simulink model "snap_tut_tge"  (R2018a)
settings: Solver=VariableStepDiscrete  StartTime=0.0  StopTime=50000  RelTol=1e-3
undefined symbols (not defined in the file): bad_frame, Bit, Both, bram, c, cnt_rst, core_rst, d, data, data_in, eof, eof_in, Falling, hex2dec, ip, ip_in, led, led_rx, led_tx, led_up, link_up, Location, Lower, Minimum_Area, notused, out, overrun, reg, Rising, ROACH2, sfp, SNAP, tx_full, tx_over, Unsigned, Upper, valid, valid_in, Width, xc7k160t
libraries: xbsIndex_r4 x1201, casper_library_misc x9, xps_library x5
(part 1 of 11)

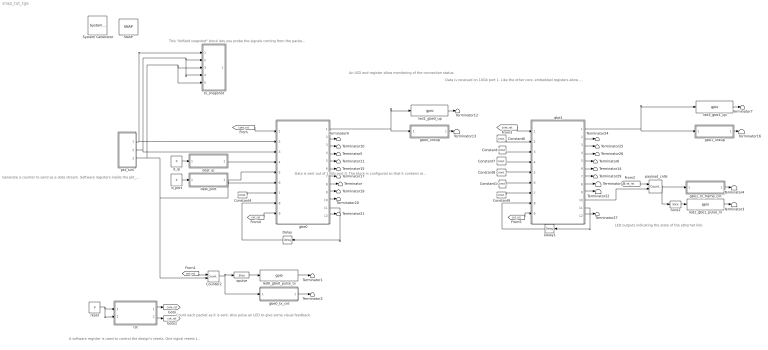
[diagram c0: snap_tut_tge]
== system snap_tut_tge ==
  note: A software register is used to control the design's resets. One signal resets the cores, the other resets the various status counters.
  note: This "bitfield snapshot" block lets you probe the signals coming from the packet simulator Using the valid signal to drive "we" and the end of frame to drive "trig" means that we can capture data starting at the beginning of a packet
  note: An LED and register allow monitoring of the connection status.
  note: Count each packet as it is sent. Also pulse an LED to give some visual feedback.
  note: LED outputs indicating the state of the ethernet link.
  note: Data is sent out of 10Gb port 0. The block is configured so that it contains all sorts of internal debug logic to count the packet rates out of, and in to, the core. The casperfpga control software knows the layout of registers inside this block, which makes it easy to grab status information
  note: Generate a counter to send as a data stream. Software registers inside the pkt_sim block allow packet sizes and counter period to be set dynamically at runtime.
  note: Data is received on 10Gb port 1. Like the other core, embedded registers allow status monitoring
  " System Generator" : xbsIndex_r4/ System Generator  Tag=genX  xilinxfamily=kintex7  part=xc7k160t  speed=-2  package=ffg676  synthesis_tool=XST  clock_wrapper=Clock Enables  directory=/home/jackh/mergeymcmergeface/tutorials_devel2/vivado/snap/tut_tge/snap_tut_tge/sysgen  proj_type=Vivado  Synth_file=Vivado Synthesis Defaults  Impl_file=Vivado Implementation Defaults  testbench=off  simulink_period=1  sysclk_period=10  dcm_input_clock_period=10  incr_netlist=off  trim_vbits=Everywhere in SubSystem  dbl_ovrd=According to Block Masks  core_generation=According to Block Masks  run_coregen=off  deprecated_control=off  eval_field=0  block_type=sysgen
  Constant : xbsIndex_r4/Constant  const=0  gui_display_data_type=Boolean  arith_type=Boolean  n_bits=16  bin_pt=14  preci_type=Single  exp_width=8  frac_width=24  explicit_period=on  period=1  equ=P=C  opselect=C  inp2=PCIN>>17  opr=+  inp1=P  carry=CIN  dbl_ovrd=off  block_type=constant
  Constant1 : xbsIndex_r4/Constant  const=0  gui_display_data_type=Boolean  arith_type=Boolean  n_bits=16  bin_pt=14  preci_type=Single  exp_width=8  frac_width=24  explicit_period=on  period=1  equ=P=C  opselect=C  inp2=PCIN>>17  opr=+  inp1=P  carry=CIN  dbl_ovrd=off  block_type=constant
  Constant4 : xbsIndex_r4/Constant  const=1  gui_display_data_type=Fixed-point  arith_type=Boolean  n_bits=1  bin_pt=0  preci_type=Single  exp_width=8  frac_width=24  explicit_period=on  period=1  equ=P=C  opselect=C  inp2=PCIN>>17  opr=+  inp1=P  carry=CIN  dbl_ovrd=off  block_type=constant
  Constant6 : xbsIndex_r4/Constant  const=0  gui_display_data_type=Fixed-point  arith_type=Unsigned  n_bits=64  bin_pt=0  preci_type=Single  exp_width=8  frac_width=24  explicit_period=on  period=1  equ=P=C  opselect=C  inp2=PCIN>>17  opr=+  inp1=P  carry=CIN  dbl_ovrd=off  block_type=constant
  Constant7 : xbsIndex_r4/Constant  const=0  gui_display_data_type=Fixed-point  arith_type=Unsigned  n_bits=32  bin_pt=0  preci_type=Single  exp_width=8  frac_width=24  explicit_period=on  period=1  equ=P=C  opselect=C  inp2=PCIN>>17  opr=+  inp1=P  carry=CIN  dbl_ovrd=off  block_type=constant
  Constant8 : xbsIndex_r4/Constant  const=0  gui_display_data_type=Fixed-point  arith_type=Unsigned  n_bits=16  bin_pt=0  preci_type=Single  exp_width=8  frac_width=24  explicit_period=on  period=1  equ=P=C  opselect=C  inp2=PCIN>>17  opr=+  inp1=P  carry=CIN  dbl_ovrd=off  block_type=constant
  Constant9 : xbsIndex_r4/Constant  const=1  gui_display_data_type=Fixed-point  arith_type=Boolean  n_bits=1  bin_pt=0  preci_type=Single  exp_width=8  frac_width=24  explicit_period=on  period=1  equ=P=C  opselect=C  inp2=PCIN>>17  opr=+  inp1=P  carry=CIN  dbl_ovrd=off  block_type=constant
  Counter2 : xbsIndex_r4/Counter  cnt_type=Free Running  cnt_to=Inf  operation=Up  start_count=0  cnt_by_val=1  arith_type=Unsigned  n_bits=32  bin_pt=0  load_pin=off  rst=on  en=on  explicit_period=on  period=1  use_behavioral_HDL=off  implementation=Fabric  dbl_ovrd=off  block_type=counter
  Delay : xbsIndex_r4/Delay  rst=off  infoeditControl=Selection of Reset will increase slice count due to use of real FFs and instead of SRLs  en=off  latency=1  reg_retiming=on  dbl_ovrd=off  block_type=delay
  Delay1 : xbsIndex_r4/Delay  rst=off  infoeditControl=Selection of Reset will increase slice count due to use of real FFs and instead of SRLs  en=off  latency=1  reg_retiming=on  dbl_ovrd=off  block_type=delay
  SNAP : xps_library/Platforms/SNAP  Tag=xps:xsg  hw_sys=SNAP:xc7k160t  clk_src=sys_clk  clk_rate=100  use_microblaze=off  sample_period=1  synthesis_tool=XST
  Slice2 : xbsIndex_r4/Slice  nbits=1  boolean_output=on  mode=Lower Bit Location + Width  bit1=0  base1=MSB of Input  bit0=27-12  base0=LSB of Input  dbl_ovrd=off  block_type=slice
  Terminator{,1..7,9..22,24..27,29} (27 alike) : Terminator
  d_ip : Constant  Value=0
  d_port : Constant  Value=0
  dest_ip : Subsystem  Tag=xps:sw_reg  AncestorBlock=xps_library/Memory/software_register  mask(swreg){io_dir=From Processor, io_delay=0, init_val=0, sample_period=1, names=reg, bitwidths=32, bin_pts=0, arith_types=0, sim_port=on, show_format=off}
      mask prompts: io_dir "I/O direction"; io_delay "I/O delay"; init_val "Initial Value"; sample_period "Sample period"; names "Bitfield names [msb...lsb]"; bitwidths "Bitfield widths"; bin_pts "Bitfield binary pts"; arith_types "Bitfield types, ufix=0, fix=1, bool=2"; sim_port "Provide sim input/output?"; show_format "Print format string?"
      mask help: A 32-bit software-accessible register. Can be divided into bitfields of varying widths and types using the fields in the block mask.
      mask init:
      | swreg_init(gcb)
  dest_port : Subsystem  Tag=xps:sw_reg  AncestorBlock=xps_library/Memory/software_register  mask(swreg){io_dir=From Processor, io_delay=0, init_val=0, sample_period=1, names=reg, bitwidths=16, bin_pts=0, arith_types=0, sim_port=on, show_format=off}
      mask prompts: io_dir "I/O direction"; io_delay "I/O delay"; init_val "Initial Value"; sample_period "Sample period"; names "Bitfield names [msb...lsb]"; bitwidths "Bitfield widths"; bin_pts "Bitfield binary pts"; arith_types "Bitfield types, ufix=0, fix=1, bool=2"; sim_port "Provide sim input/output?"; show_format "Print format string?"
      mask help: A 32-bit software-accessible register. Can be divided into bitfields of varying widths and types using the fields in the block mask.
      mask init:
      | swreg_init(gcb)
  gbe0 : Subsystem  Tag=xps:ten_gbe  AncestorBlock=xps_library/IO/ten_gbe  mask(ten_gbe){flavour=sfp+, slot=0, port_r1=0, port_r2_cx4=0, port_r2_sfpp=0, rx_dist_ram=off, large_frames=on, show_param=off, pre_emph_r2=1.07, pre_emph=3, post_emph_r2=0.18, rxeqmix_r2=7, swing_r2=940, swing=800, fab_en=on, fab_mac=hex2dec('123456780000'), fab_ip=192*(2^24) + 168*(2^16) + 5*(2^8) + 20*(2^0), fab_udp=10000, fab_gate=1, cpu_rx_en=on, cpu_tx_en=on, ttl=hex2dec('FF'), promisc_mode=off, debug_ctr_width=32, txctr=on, txerrctr=off, txerrctr_len=100, txofctr=on, txfullctr=on, txvldctr=on, txsnaplen=8192, rxctr=on, rxerrctr=off, rxerrctr_len=100, rxofctr=on, rxbadctr=on, rxvldctr=on, rxeofctr=on, rxsnaplen=8192}
      mask prompts: flavour "Mezzanine card flavour"; slot "Card slot"; port_r1 "Port"; port_r2_cx4 "Port"; port_r2_sfpp "Port"; rx_dist_ram "Shallow RX Fifo (Beware overruns!)"; large_frames "Enable Large TX Frames (8k+512)"; show_param "---------------------- Show Implementation Parameters -----------------------------------------------------------------------------------"; pre_emph_r2 "Pre-emphasis (dB)"; pre_emph "Pre-emphasis"; post_emph_r2 "Post-emphasis (dB)"; rxeqmix_r2 "Receive equalisation"; swing_r2 "Driver Swing Control (mVppd)"; swing "Differential swing"; fab_en "Enable fabric on startup"; fab_mac "Fabric MAC Address"; fab_ip "Fabric IP Address"; fab_udp "Fabric UDP Port"; fab_gate "Fabric Gateway"; cpu_rx_en "Enable CPU RX"; cpu_tx_en "Enable CPU TX"; promisc_mode "Promiscuous mode"; debug_ctr_width "Debug counter width"; txctr "TX - core_txctr"; txerrctr "TX packet length error - core_txerrctr"; txerrctr_len "-- expected TX packet length"; txofctr "TX overflow - core_txofctr"; txfullctr "TX full - core_txfullctr"; txvldctr "TX valid cycle - core_txvldctr"; txsnaplen "TX snapshot length"; rxctr "RX - core_rxctr"; rxerrctr "RX packet length error - core_rxerrctr"; rxerrctr_len "-- expected RX packet length"; rxofctr "RX overflow - core_rxofctr"; rxbadctr "RX bad - core_rxbadctr"; rxvldctr "RX valid cycle - core_rxvldctr"; rxeofctr "RX eof - core_rxeofctr"; rxsnaplen "RX snapshot length"
      mask help: This block sends and receives UDP frames (packets). It accepts a 64 bit wide data stream with user-determined frame breaks. The data stream is wrapped in a UDP frame for transmission. Incoming UDP packets are unwrapped and the data presented as a 64 bit wide stream.
      mask init:
      | temp = eval(get_param(gcb, 'debug_ctr_width'));
      | if temp <= 0,
      |     error('Debug counters cannot be ltoet zero.');
      | end
      | tengbe_mask(gcb)
  gbe0_linkup : Subsystem  Tag=xps:sw_reg  AncestorBlock=xps_library/Memory/software_register  mask(swreg){io_dir=To Processor, io_delay=0, init_val=0, sample_period=1, names=reg, bitwidths=1, bin_pts=0, arith_types=2, sim_port=on, show_format=off}
      mask prompts: io_dir "I/O direction"; io_delay "I/O delay"; init_val "Initial Value"; sample_period "Sample period"; names "Bitfield names [msb...lsb]"; bitwidths "Bitfield widths"; bin_pts "Bitfield binary pts"; arith_types "Bitfield types, ufix=0, fix=1, bool=2"; sim_port "Provide sim input/output?"; show_format "Print format string?"
      mask help: A 32-bit software-accessible register. Can be divided into bitfields of varying widths and types using the fields in the block mask.
      mask init:
      | swreg_init(gcb)
  gbe0_tx_cnt : Subsystem  Tag=xps:sw_reg  AncestorBlock=xps_library/Memory/software_register  mask(swreg){io_dir=To Processor, io_delay=0, init_val=0, sample_period=1, names=reg, bitwidths=32, bin_pts=0, arith_types=0, sim_port=on, show_format=off}
      mask prompts: io_dir "I/O direction"; io_delay "I/O delay"; init_val "Initial Value"; sample_period "Sample period"; names "Bitfield names [msb...lsb]"; bitwidths "Bitfield widths"; bin_pts "Bitfield binary pts"; arith_types "Bitfield types, ufix=0, fix=1, bool=2"; sim_port "Provide sim input/output?"; show_format "Print format string?"
      mask help: A 32-bit software-accessible register. Can be divided into bitfields of varying widths and types using the fields in the block mask.
      mask init:
      | swreg_init(gcb)
  gbe1 : Subsystem  Tag=xps:ten_gbe  AncestorBlock=xps_library/IO/ten_gbe  mask(ten_gbe){flavour=sfp+, slot=0, port_r1=1, port_r2_cx4=0, port_r2_sfpp=0, rx_dist_ram=off, large_frames=on, show_param=on, pre_emph_r2=1.07, pre_emph=3, post_emph_r2=0.18, rxeqmix_r2=7, swing_r2=940, swing=800, fab_en=on, fab_mac=hex2dec('123456780001'), fab_ip=192*(2^24) + 168*(2^16) + 5*(2^8) + 21*(2^0), fab_udp=10000, fab_gate=1, cpu_rx_en=on, cpu_tx_en=on, ttl=hex2dec('FF'), promisc_mode=off, debug_ctr_width=32, txctr=on, txerrctr=off, txerrctr_len=100, txofctr=on, txfullctr=on, txvldctr=on, txsnaplen=8192, rxctr=on, rxerrctr=off, rxerrctr_len=100, rxofctr=on, rxbadctr=on, rxvldctr=on, rxeofctr=on, rxsnaplen=8192}
      mask prompts: flavour "Mezzanine card flavour"; slot "Card slot"; port_r1 "Port"; port_r2_cx4 "Port"; port_r2_sfpp "Port"; rx_dist_ram "Shallow RX Fifo (Beware overruns!)"; large_frames "Enable Large TX Frames (8k+512)"; show_param "---------------------- Show Implementation Parameters -----------------------------------------------------------------------------------"; pre_emph_r2 "Pre-emphasis (dB)"; pre_emph "Pre-emphasis"; post_emph_r2 "Post-emphasis (dB)"; rxeqmix_r2 "Receive equalisation"; swing_r2 "Driver Swing Control (mVppd)"; swing "Differential swing"; fab_en "Enable fabric on startup"; fab_mac "Fabric MAC Address"; fab_ip "Fabric IP Address"; fab_udp "Fabric UDP Port"; fab_gate "Fabric Gateway"; cpu_rx_en "Enable CPU RX"; cpu_tx_en "Enable CPU TX"; promisc_mode "Promiscuous mode"; debug_ctr_width "Debug counter width"; txctr "TX - core_txctr"; txerrctr "TX packet length error - core_txerrctr"; txerrctr_len "-- expected TX packet length"; txofctr "TX overflow - core_txofctr"; txfullctr "TX full - core_txfullctr"; txvldctr "TX valid cycle - core_txvldctr"; txsnaplen "TX snapshot length"; rxctr "RX - core_rxctr"; rxerrctr "RX packet length error - core_rxerrctr"; rxerrctr_len "-- expected RX packet length"; rxofctr "RX overflow - core_rxofctr"; rxbadctr "RX bad - core_rxbadctr"; rxvldctr "RX valid cycle - core_rxvldctr"; rxeofctr "RX eof - core_rxeofctr"; rxsnaplen "RX snapshot length"
      mask help: This block sends and receives UDP frames (packets). It accepts a 64 bit wide data stream with user-determined frame breaks. The data stream is wrapped in a UDP frame for transmission. Incoming UDP packets are unwrapped and the data presented as a 64 bit wide stream.
      mask init:
      | temp = eval(get_param(gcb, 'debug_ctr_width'));
      | if temp <= 0,
      |     error('Debug counters cannot be ltoet zero.');
      | end
      | tengbe_mask(gcb)
  gbe1_linkup : Subsystem  Tag=xps:sw_reg  AncestorBlock=xps_library/Memory/software_register  mask(swreg){io_dir=To Processor, io_delay=0, init_val=0, sample_period=1, names=reg, bitwidths=1, bin_pts=0, arith_types=2, sim_port=on, show_format=off}
      mask prompts: io_dir "I/O direction"; io_delay "I/O delay"; init_val "Initial Value"; sample_period "Sample period"; names "Bitfield names [msb...lsb]"; bitwidths "Bitfield widths"; bin_pts "Bitfield binary pts"; arith_types "Bitfield types, ufix=0, fix=1, bool=2"; sim_port "Provide sim input/output?"; show_format "Print format string?"
      mask help: A 32-bit software-accessible register. Can be divided into bitfields of varying widths and types using the fields in the block mask.
      mask init:
      | swreg_init(gcb)
  gbe1_rx_frame_cnt : Subsystem  Tag=xps:sw_reg  AncestorBlock=xps_library/Memory/software_register  mask(swreg){io_dir=To Processor, io_delay=0, init_val=0, sample_period=1, names=reg, bitwidths=32, bin_pts=0, arith_types=0, sim_port=on, show_format=off}
      mask prompts: io_dir "I/O direction"; io_delay "I/O delay"; init_val "Initial Value"; sample_period "Sample period"; names "Bitfield names [msb...lsb]"; bitwidths "Bitfield widths"; bin_pts "Bitfield binary pts"; arith_types "Bitfield types, ufix=0, fix=1, bool=2"; sim_port "Provide sim input/output?"; show_format "Print format string?"
      mask help: A 32-bit software-accessible register. Can be divided into bitfields of varying widths and types using the fields in the block mask.
      mask init:
      | swreg_init(gcb)
  led0_gbe0_pulse_tx : xps_library/IO/gpio  Tag=xps:gpio  io_group_params_forwarded=on  io_group=ROACH2:led  io_group_real=led  io_group_custom=0  io_dir=out  arith_type=Boolean  bitwidth=1  bin_pt=0  bit_index=0  sample_period=1  use_single_ended=off  use_ddr=off  reg_iob=on  reg_clk_phase=0  termination=None
  led1_gbe0_up : xps_library/IO/gpio  Tag=xps:gpio  io_group_params_forwarded=on  io_group=ROACH2:led  io_group_real=led  io_group_custom=0  io_dir=out  arith_type=Boolean  bitwidth=1  bin_pt=0  bit_index=1  sample_period=1  use_single_ended=off  use_ddr=off  reg_iob=on  reg_clk_phase=0  termination=None
  led2_gbe1_pulse_rx : xps_library/IO/gpio  Tag=xps:gpio  io_group_params_forwarded=on  io_group=ROACH2:led  io_group_real=led  io_group_custom=0  io_dir=out  arith_type=Boolean  bitwidth=1  bin_pt=0  bit_index=2  sample_period=1  use_single_ended=off  use_ddr=off  reg_iob=off  reg_clk_phase=0  termination=None
  led3_gbe1_up : xps_library/IO/gpio  Tag=xps:gpio  io_group_params_forwarded=on  io_group=ROACH2:led  io_group_real=led  io_group_custom=0  io_dir=out  arith_type=Boolean  bitwidth=2  bin_pt=0  bit_index=3  sample_period=1  use_single_ended=off  use_ddr=off  reg_iob=on  reg_clk_phase=0  termination=None
  payload_cnt6 : xbsIndex_r4/Counter  cnt_type=Free Running  cnt_to=0  operation=Up  start_count=0  cnt_by_val=1  arith_type=Unsigned  n_bits=32  bin_pt=0  load_pin=off  rst=on  en=on  explicit_period=on  period=1  use_behavioral_HDL=off  implementation=Fabric  use_rpm=on  dbl_ovrd=off  block_type=counter
  pkt_sim : Subsystem
  reset : Constant  Value=0
  rst : Subsystem  Tag=xps:sw_reg  AncestorBlock=xps_library/Memory/software_register  mask(swreg){io_dir=From Processor, io_delay=0, init_val=0, sample_period=1, names=[core_rst cnt_rst], bitwidths=[1 1], bin_pts=0, arith_types=[2 2], sim_port=on, show_format=off}
      mask prompts: io_dir "I/O direction"; io_delay "I/O delay"; init_val "Initial Value"; sample_period "Sample period"; names "Bitfield names [msb...lsb]"; bitwidths "Bitfield widths"; bin_pts "Bitfield binary pts"; arith_types "Bitfield types, ufix=0, fix=1, bool=2"; sim_port "Provide sim input/output?"; show_format "Print format string?"
      mask help: A 32-bit software-accessible register. Can be divided into bitfields of varying widths and types using the fields in the block mask.
      mask init:
      | swreg_init(gcb)
  spulse : xbsIndex_r4/Slice  nbits=1  boolean_output=on  mode=Lower Bit Location + Width  bit1=0  base1=MSB of Input  bit0=27-12  base0=LSB of Input  dbl_ovrd=off  block_type=slice
  tx_snapshot : Subsystem  Tag=casper:bitsnap  AncestorBlock=casper_library_scopes/bitfield_snapshot  mask(bitsnap){io_names=[data valid eof], io_widths=[64 1 1], io_bps=[0 0 0], io_types=[0 2 2], show_format=on, snap_storage=bram, snap_dram_dimm=2, snap_dram_clock=250, snap_nsamples=12, snap_data_width=128, snap_offset=off, snap_circap=off, snap_value=off, snap_ext_arm=off, snap_ext_circ=off, snap_provide_outputs=on, snap_use_dsp48=on, snap_delay=0, extra_names=[c d], extra_widths=[30 2], extra_bps=[0 0], extra_types=[0 0]}
      mask prompts: io_names "Names [msb...lsb]"; io_widths "Bitwidths [msb...lsb]"; io_bps "Binary pts [msb...lsb]"; io_types "Data types [msb...lsb], ufix=0, fix=1, bool=2"; show_format "Print format string?"; snap_storage "Storage medium"; snap_dram_dimm "DRAM dimm"; snap_dram_clock "DRAM clock rate"; snap_nsamples "Number of Samples (2^?)"; snap_data_width "Data width"; snap_offset "Start delay support"; snap_circap "Circular capture support"; snap_value "Extra value capture support"; snap_ext_arm "External arm support"; snap_ext_circ "External circular capture support"; snap_provide_outputs "Provide outputs"; snap_use_dsp48 "Use DSP48s to implement counters"; snap_delay "Pre-snapshot delay"; extra_names "Names [msb...lsb]"; extra_widths "Widths [msb...lsb]"; extra_bps "Binary pts [msb...lsb]"; extra_types "Data types [msb...lsb], ufix=0, fix=1, bool=2"
      mask help: A wrapped snapshot block. Allows specification of inputs to a snapblock word so the toolflow can automatically set up the scope. See documentation for snapshot for explanation of parameters.
      mask init:
      | bitsnap_init(gcb);
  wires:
  reset/1 -> rst/2(sim_2), rst/1(sim_1)
  rst/2(in_cnt_rst) -> [cnt_rst]
  rst/1(in_core_rst) -> [core_rst]
  dest_ip/1(in_reg) -> gbe0/4(tx_dest_ip)
  dest_port/1(in_reg) -> gbe0/5(tx_dest_port)
  d_ip/1 -> dest_ip/1(sim_1)
  d_port/1 -> dest_port/1(sim_1)
  [core_rst] -> gbe0/1(rst)
  pkt_sim/1(d_out) -> gbe0/2(tx_data), tx_snapshot/1(in_data)
  Constant4/1 -> gbe0/7(rx_ack)
  gbe0/11(rx_bad_frame) -> Delay/1
  gbe0/8(rx_source_ip) -> Terminator/1
  Delay/1 -> gbe0/8(rx_overrun_ack)
  spulse/1 -> led0_gbe0_pulse_tx/1
  Counter2/1 -> spulse/1, gbe0_tx_cnt/1(out_reg)
  [cnt_rst] -> Counter2/1
  led0_gbe0_pulse_tx/1 -> Terminator1/1
  gbe0_tx_cnt/1(sim_out) -> Terminator2/1
  gbe0_linkup/1(sim_out) -> Terminator13/1
  [cnt_rst] -> payload_cnt6/1
  Constant6/1 -> gbe1/2(tx_data)
  Constant/1 -> gbe1/3(tx_valid)
  Constant7/1 -> gbe1/4(tx_dest_ip)
  Constant8/1 -> gbe1/5(tx_dest_port)
  Constant1/1 -> gbe1/6(tx_end_of_frame)
  Constant9/1 -> gbe1/7(rx_ack)
  gbe1/11(rx_bad_frame) -> Delay1/1
  Delay1/1 -> gbe1/8(rx_overrun_ack)
  payload_cnt6/1 -> gbe1_rx_frame_cnt/1(out_reg), Slice2/1
  Slice2/1 -> led2_gbe1_pulse_rx/1
  [core_rst] -> gbe1/1(rst)
  gbe1_rx_frame_cnt/1(sim_out) -> Terminator4/1
  led2_gbe1_pulse_rx/1 -> Terminator3/1
  gbe1_linkup/1(sim_out) -> Terminator16/1
  gbe1/8(rx_source_ip) -> Terminator18/1
  gbe0/1(led_up) -> led1_gbe0_up/1, gbe0_linkup/1(out_reg)
  led1_gbe0_up/1 -> Terminator12/1
  led3_gbe1_up/1 -> Terminator7/1
  gbe1/1(led_up) -> gbe1_linkup/1(out_reg), led3_gbe1_up/1
  gbe0/2(led_rx) -> Terminator9/1
  gbe0/3(led_tx) -> Terminator10/1
  gbe0/5(tx_overflow) -> Terminator11/1
  gbe0/6(rx_data) -> Terminator15/1
  gbe0/7(rx_valid) -> Terminator17/1
  gbe0/9(rx_source_port) -> Terminator19/1
  gbe0/10(rx_end_of_frame) -> Terminator20/1
  gbe0/12(rx_overrun) -> Terminator21/1
  gbe1/2(led_rx) -> Terminator24/1
  gbe1/3(led_tx) -> Terminator25/1
  gbe1/4(tx_afull) -> Terminator26/1
  gbe1/12(rx_overrun) -> Terminator27/1
  [cnt_rst] -> gbe0/9(debug_rst)
  [cnt_rst] -> gbe1/9(debug_rst)
  gbe0/4(tx_afull) -> Terminator5/1
  gbe1/5(tx_overflow) -> Terminator6/1
  gbe1/6(rx_data) -> Terminator14/1
  gbe1/7(rx_valid) -> Terminator29/1
  gbe1/10(rx_end_of_frame) -> payload_cnt6/2
  gbe1/9(rx_source_port) -> Terminator22/1
  pkt_sim/3(eof) -> tx_snapshot/5(trig), tx_snapshot/3(in_eof), gbe0/6(tx_end_of_frame), Counter2/2
  pkt_sim/2(valid) -> gbe0/3(tx_valid), tx_snapshot/4(we), tx_snapshot/2(in_valid)

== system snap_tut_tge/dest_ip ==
  sim_1 : Inport
  convert1_1 : DataTypeConversion  OutDataTypeStr=fixdt('ufix32_En0')
  convert2_1 : DataTypeConversion  OutDataTypeStr=fixdt('ufix32_En0')  ConvertRealWorld=Stored Integer (SI)
  gain_1 : Gain
  io_delay : xbsIndex_r4/Delay  rst=off  infoeditControl=Selection of Reset will increase slice count due to use of real FFs and instead of SRLs  en=off  latency=0  reg_retiming=on  dbl_ovrd=off  block_type=delay
  reint1 : xbsIndex_r4/Reinterpret  force_arith_type=on  arith_type=Unsigned  force_bin_pt=on  bin_pt=0  block_type=reinterpret
  slice_reg : xbsIndex_r4/Slice  nbits=32  boolean_output=off  mode=Lower Bit Location + Width  bit1=0  base1=MSB of Input  bit0=0  base0=LSB of Input  dbl_ovrd=off  block_type=slice
  snap_tut_tge_dest_ip_user_data_out : xbsIndex_r4/Gateway In  gui_display_data_type=Fixed-point  arith_type=Unsigned  n_bits=32  bin_pt=0  preci_type=Single  exp_width=8  frac_width=24  rows=1  columns=1  quantization="Round  (unbiased: +/- Inf)"  overflow=Saturate  period=1  UseAsADC=off  ADCChannel='1'  interface=None  automatic_assignment=on  address_offset=hex2dec('00')  intf_name=''  intf_description=''  default_value=0  timing_constraint=None  locs_specified=off  LOCs={}  io_standard={}  inherit_from_input=off  hdl_port=on  dbl_ovrd=off  block_type=gatewayin
  in_reg : Outport
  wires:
  snap_tut_tge_dest_ip_user_data_out/1 -> io_delay/1
  sim_1/1 -> convert1_1/1
  convert1_1/1 -> convert2_1/1
  convert2_1/1 -> gain_1/1
  gain_1/1 -> snap_tut_tge_dest_ip_user_data_out/1
  io_delay/1 -> slice_reg/1
  slice_reg/1 -> reint1/1
  reint1/1 -> in_reg/1

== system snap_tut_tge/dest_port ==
  sim_1 : Inport
  convert1_1 : DataTypeConversion  OutDataTypeStr=fixdt('ufix16_En0')
  convert2_1 : DataTypeConversion  OutDataTypeStr=fixdt('ufix16_En0')  ConvertRealWorld=Stored Integer (SI)
  gain_1 : Gain
  io_delay : xbsIndex_r4/Delay  rst=off  infoeditControl=Selection of Reset will increase slice count due to use of real FFs and instead of SRLs  en=off  latency=0  reg_retiming=on  dbl_ovrd=off  block_type=delay
  reint1 : xbsIndex_r4/Reinterpret  force_arith_type=on  arith_type=Unsigned  force_bin_pt=on  bin_pt=0  block_type=reinterpret
  slice_reg : xbsIndex_r4/Slice  nbits=16  boolean_output=off  mode=Lower Bit Location + Width  bit1=0  base1=MSB of Input  bit0=0  base0=LSB of Input  dbl_ovrd=off  block_type=slice
  snap_tut_tge_dest_port_user_data_out : xbsIndex_r4/Gateway In  gui_display_data_type=Fixed-point  arith_type=Unsigned  n_bits=32  bin_pt=0  preci_type=Single  exp_width=8  frac_width=24  rows=1  columns=1  quantization="Round  (unbiased: +/- Inf)"  overflow=Saturate  period=1  UseAsADC=off  ADCChannel='1'  interface=None  automatic_assignment=on  address_offset=hex2dec('00')  intf_name=''  intf_description=''  default_value=0  timing_constraint=None  locs_specified=off  LOCs={}  io_standard={}  inherit_from_input=off  hdl_port=on  dbl_ovrd=off  block_type=gatewayin
  in_reg : Outport
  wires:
  snap_tut_tge_dest_port_user_data_out/1 -> io_delay/1
  sim_1/1 -> convert1_1/1
  convert1_1/1 -> convert2_1/1
  convert2_1/1 -> gain_1/1
  gain_1/1 -> snap_tut_tge_dest_port_user_data_out/1
  io_delay/1 -> slice_reg/1
  slice_reg/1 -> reint1/1
  reint1/1 -> in_reg/1
